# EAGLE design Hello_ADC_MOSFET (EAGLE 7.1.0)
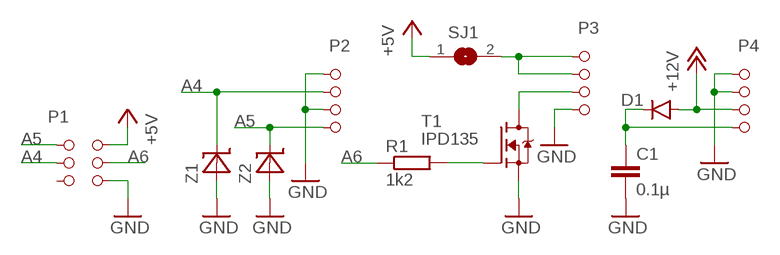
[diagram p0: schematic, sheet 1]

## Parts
C1  0.1µ  C-EUC1206  [C1206]
D1  DIODESMA-KIT  [SMA-DIODE-KIT]
P1  SMD-3-2  [SMD-3-2]
P2  SMD-2-2  [SMD-2-2]
P3  SMD-2-2  [SMD-2-2]
P4  SMD-2-2  [SMD-2-2]
R1  1k2  R-EU_R1206  [R1206]
SJ1  SJ  [SJ]
T1  IPD135  IPD135N03L  [DPACK]
Z1  3v3  ZENER-SOD123SOD-123  [SOD123]
Z2  3v3  ZENER-SOD123SOD-123  [SOD123]

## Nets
+5V: P1.1 SJ1.1
+12V: D1.A P4.3
A4: P1.5 P2.2 Z1.C
A5: P1.6 P2.4 Z2.C
A6: P1.2 R1.1
GND: C1.2 P1.3 P2.1 P2.3 P3.4 P4.1 P4.2 T1.S Z1.A Z2.A
N$1: R1.2 T1.G
N$2: P3.3 T1.D
N$3: P3.1 P3.2 SJ1.2
N$4: C1.1 D1.C P4.4
Unconnected: P1.4

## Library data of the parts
C1 = rcl:C-EU: CAPACITOR, European symbol
D1 = SparkFun-DiscreteSemi:DIODE: Diode
P1 = PinHeader:SMD-3-2
P2-P4 = PinHeader:SMD-2-2
R1 = rcl:R-EU_: RESISTOR, European symbol
SJ1 = jumper:SJ: SMD solder JUMPER
T1 = MOSFET:IPD135N03L
Z1 Z2 = diode:ZENER-SOD123

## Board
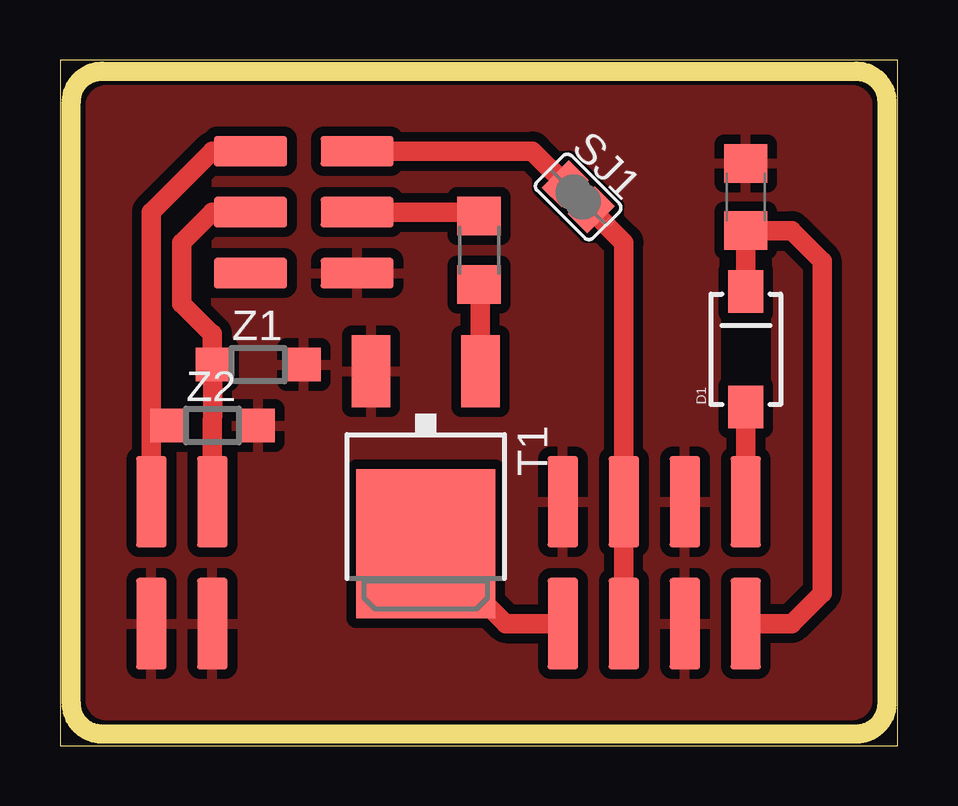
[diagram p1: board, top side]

Size 34.91 x 28.57 mm. Coordinates in mm from the lower left corner, seen from the top.
Outline: 0,0 34.91,0 34.91,28.57 0,28.57 0,0
Copper layers (1*16): Top 0.035mm / dielectric 1.5mm / Bottom 0.035mm
Design rules "default *": minimum track width 10mil, minimum drill 24mil, track to track 8mil, track to pad 8mil, pad to pad 8mil, via to via 8mil, smd to smd 8mil, copper to edge 40mil, drill to drill 8mil, minimum pad ring 10mil, minimum via ring 8mil, stop-mask expansion 4mil, vias tented up to drill 0mil, thermal gap 16mil
tRestrict: area 27.9,15.2 to 29.2,17.8
Milling: 8 lines

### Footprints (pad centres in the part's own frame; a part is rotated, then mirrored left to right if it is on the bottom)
C1206 = smd 1.6 x 1.8: 1 -1.4,0; 2 1.4,0
SMA-DIODE-KIT = smd 1.77 x 1.47: A -2.4,0; C 2.4,0
SMD-3-2 = smd 1.27 x 3.048: 1 -2.54,2.223; 2 0,2.223; 3 2.54,2.223; 4 2.54,-2.223; 5 0,-2.223; 6 -2.54,-2.223
SMD-2-2 = smd 1.27 x 3.81: 1 -1.27,2.54; 2 -1.27,-2.54; 3 1.27,2.54; 4 1.27,-2.54
R1206 = smd 1.6 x 1.803: 1 -1.422,0; 2 1.422,0
SJ = smd 1.168 x 1.6: 1 -0.762,0; 2 0.762,0
DPACK = smd 5.8 x 6.2: D 0,1.11 | smd 1.6 x 3: G -2.28,-6.07; S 2.28,-6.07
SOD123 = smd 1.4 x 1.4: A 1.9,0; C -1.9,0

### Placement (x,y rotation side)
C1  28.57,22.86 90 top
D1  28.57,16.51 90 top
P1  10.16,22.23 270 top
P2  5.08,7.62 180 top
P3  22.23,7.62 180 top
P4  27.3,7.62 0 top
R1  17.46,20.64 270 top
SJ1  21.59,22.86 315 top
T1  15.24,9.53 180 top
Z1  8.26,15.88 0 top
Z2  6.35,13.34 0 top

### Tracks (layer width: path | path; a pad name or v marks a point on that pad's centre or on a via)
+5V
  Top 0.813: P1.1 19.68,24.77 SJ1.1
+12V
  Top 0.813: D1.A P4.3
A4
  Top 0.813: P2.2 6.35,11.43 Z1.C 6.35,17.15 6.35,17.14 5.08,18.41 5.08,20.95 6.35,22.23 P1.5
A5
  Top 0.813: P1.6 6.35,24.77 3.81,22.23 3.81,13.34 | 3.81,13.34 P2.4 | Z2.C 3.81,13.34
A6
  Top 0.813: P1.2 17.3,22.23 R1.1
GND
  pour Top (isolate 0.406): 1.27,26.67 1.27,1.91 arc90 1.91,1.27 33.02,1.27 arc90 33.66,1.91 33.66,26.67 arc90 33.02,27.3 1.91,27.3 arc90
N$1
  Top 0.813: T1.G 17.52,19.16 R1.2
N$2
  Top 0.813: T1.D 18.57,5.08 P3.3
N$3
  Top 0.813: P3.1 P3.2 23.5,20.95 SJ1.2
N$4
  Top 0.813: D1.C C1.1 30.48,21.46 31.75,20.19 31.75,6.35 30.48,5.08 P4.4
